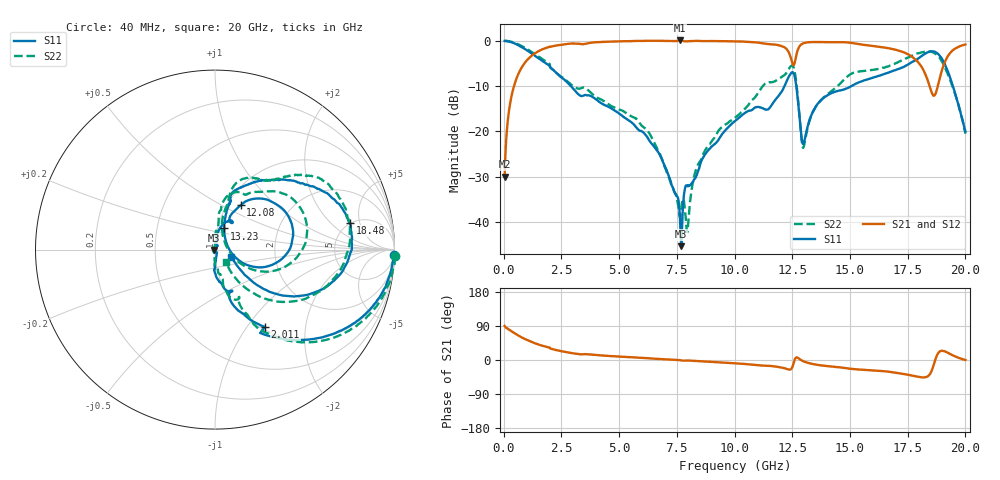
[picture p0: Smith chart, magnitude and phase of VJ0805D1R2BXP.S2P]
! VJ0805D1R2BXP
! DATE 10/29/2021  11:28
! CAPACITORS MOUNTED IN SERIES ON 25 MIL THICK MICROSTRIP SUBSTRATE
# GHz  S  MA  R  50.00
!  FREQ  S11M  S11A  S21M  S21A  S12M  S12A  S22M  S22A
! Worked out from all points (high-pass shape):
!   1601 points, 40 MHz to 20 GHz, reference 50 ohm
!   highest |S21| = 0.08 dB at 7.65 GHz (marker M1); lowest = -30.0 dB at 40 MHz (marker M2)
!   |S21| within 3 dB of the highest: 1.306 GHz to 12.38 GHz (11.07 GHz wide, 162 % of centre); 12.69 GHz to 17.49 GHz (4.804 GHz wide, 31.8 % of centre)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
!   lowest |S11| = -45.4 dB at 7.687 GHz (marker M3), VSWR 1.01, Z = 49.5 - j0.223 ohm
!   |S11| at or under -10 dB: 2.911 GHz to 12.16 GHz (9.254 GHz wide, 123 % of centre); 12.67 GHz to 15.06 GHz (2.384 GHz wide, 17.2 % of centre); 19.46 GHz to end of sweep
!   |S22| runs from -42.3 to 0.0 dB; largest |S21 - S12| = 0.0056
!   S11 on the Smith chart (normalised r, x): 40 MHz: 8, -63; 2.011 GHz: 1.04, -1.22; 12.08 GHz: 1.15, +0.62; 13.23 GHz: 1.08, +0.26; 18.48 GHz: 4.91, +3.55; 20 GHz: 1.20, -0.10
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0.04  0.9958 -1.8  0.03147 89.7  0.02782 89.1  1.003 -2.1
0.252075  0.9768 -10.7  0.1846 79.1  0.1847 79.1  0.989 -10.8
0.56395  0.914 -22.9  0.3897 67.1  0.3891 67.3  0.931 -23.1
2.01105  0.5129 -57.2  0.8567 30.4  0.8557 30.4  0.507 -61.2
3.370825  0.245 -68.6  0.9198 15.0  0.9179 15.0  0.3005 -63.1
6.70165  0.05851 -84.8  1 2.8  0.9988 2.7  0.06079 -91.8
7.64975  0.008866 -102.5  1.01 -0.5  1.009 -0.6  0.01154 147.5
7.687175  0.005386 -155.3  1.009 -1.0  1.007 -1.1  0.01362 108.5
7.911725  0.02509 56.7  0.9862 -1.4  0.9845 -1.5  0.008976 27.8
8.410725  0.03585 77.9  0.9979 -3.0  0.9962 -3.2  0.04258 84.8
10.02  0.1299 75.0  0.9861 -8.7  0.9842 -8.8  0.1417 82.4
12.07837  0.2849 60.0  0.8671 -20.4  0.8657 -20.5  0.4048 52.7
12.5649  0.4346 7.3  0.539 -7.3  0.5387 -7.4  0.5042 3.9
12.9641  0.07254 19.2  0.9356 -2.8  0.934 -2.9  0.06606 20.0
13.22607  0.1285 66.5  0.9647 -8.4  0.9635 -8.4  0.1253 72.2
13.35083  0.1567 70.1  0.9679 -10.2  0.9674 -10.3  0.1547 75.6
15.01  0.3104 73.8  0.9519 -23.0  0.9513 -23.1  0.4258 68.1
16.68165  0.4479 58.0  0.8268 -31.0  0.8255 -31.2  0.5241 48.7
17.8044  0.6028 37.7  0.6309 -42.6  0.6291 -42.6  0.7076 33.8
18.47805  0.7662 11.2  0.3002 -35.8  0.2987 -36.0  0.7593 8.1
19.1018  0.556 -27.4  0.5752 22.9  0.5744 22.8  0.5171 -34.0
20  0.09972 -24.1  0.9104 -0.0  0.9094 -0.1  0.09419 -48.6
